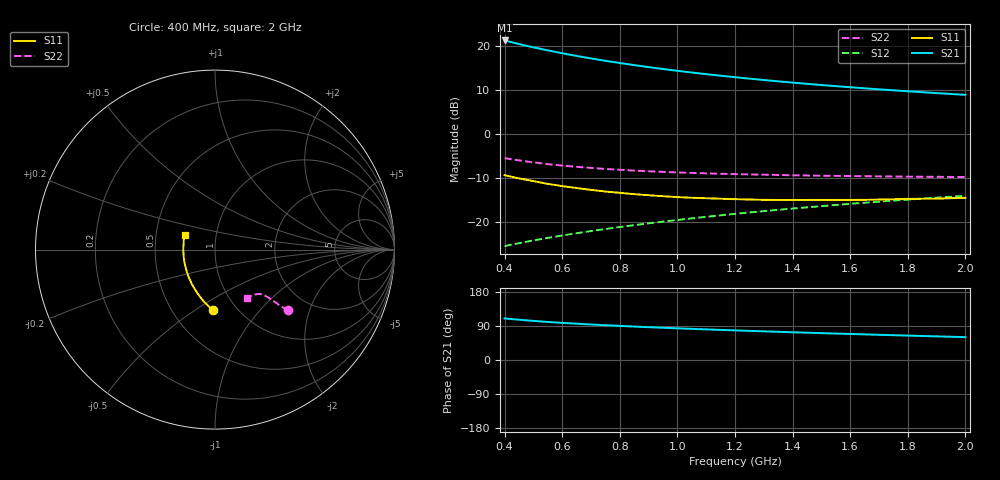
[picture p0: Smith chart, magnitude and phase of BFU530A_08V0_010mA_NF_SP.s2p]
! Filename:  P:\Prog\Test\Noise\ATS_data\Testdata_Net\06 Compressed Noise after Statistics\BFU530A_APG2013_33_A05_08p0V_010mA_NF_CM01_D.sf
! Date/Time: Tue 16/Apr/2013 15:11:01
! BFU530A_APG2013_33_A05_08p0V_1to25mA_NF_CM01_Bias5_R.sf
! Noise Parameter Data File
! BFU530A_APG2013_33_A05_08p0V_1to25mA_NF_CM01
! Date/time: Fri Apr 12 16:45:05 2013
! VAR V_out= 8.001000
! VAR I_out= 9.995000
! VAR V_in= 0.820500
! VAR I_in= 0.102910
! Device data file deembeded for feedlines and parallel
! Original file: \06 Compressed Noise after Statistics\BFU530A_APG2013_33_A05_08p0V_010mA_NF_CM01_R.sf
! Feed-files: PR017V01_150413_Feed1.s2p, PR017V01_150413_Feed2.s2p
! Parallel-file: PR017V01_150413_Par.s2p
# MHz S MA R 50
!  Freq-MHz  S11-mag  S11-arg  S21-mag  S21-arg  S12-mag  S12-arg  S22-mag  S22-arg
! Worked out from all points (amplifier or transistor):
!   37 points, 400 MHz to 2 GHz, reference 50 ohm
!   highest |S21| = 21.3 dB at 400 MHz (marker M1)
!   |S21| within 3 dB of that: start of sweep to 606.9 MHz
!   unconditionally stable (mu >= 1): 1.335 GHz to end of sweep
!   at 500 MHz: K = 0.80, MSG = 22.0 dB, |S12| = -24.3 dB
!   at 1.1 GHz: K = 0.98, MSG = 16.2 dB, |S12| = -18.9 dB
!   at 2 GHz: K = 1.01, MAG = 11.0 dB, |S12| = -14.1 dB
!   lowest NFmin = 0.76 dB at 433 MHz
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400  0.3384 -91.7  11.59 109.8  0.05265 65.0  0.5294 -39.6
420  0.3274 -94.2  11.16 108.3  0.05443 65.0  0.5163 -39.9
440  0.3163 -96.8  10.75 106.9  0.0561 65.1  0.5048 -40.1
480  0.2984 -101.5  10.01 104.4  0.05948 65.3  0.4836 -40.6
500  0.2896 -103.8  9.673 103.2  0.06122 65.4  0.4745 -40.8
550  0.2696 -109.5  8.942 100.4  0.06535 65.7  0.4523 -41.1
600  0.2544 -114.5  8.287 98.0  0.06966 66.0  0.4359 -41.3
650  0.2418 -119.4  7.727 95.8  0.07396 66.3  0.422 -41.6
700  0.2304 -124.1  7.235 93.7  0.07826 66.6  0.4098 -41.8
750  0.2207 -128.6  6.798 91.8  0.08259 66.9  0.399 -42.0
800  0.2134 -133.1  6.416 90.0  0.087 67.1  0.3905 -42.2
850  0.206 -137.5  6.072 88.3  0.09137 67.3  0.3821 -42.5
900  0.2003 -141.6  5.763 86.6  0.0958 67.4  0.3751 -42.8
950  0.1952 -145.5  5.484 85.1  0.1002 67.5  0.3695 -43.2
1050  0.1874 -153.0  5 82.2  0.1092 67.7  0.3595 -43.8
1150  0.1828 -160.3  4.598 79.4  0.1182 67.7  0.3513 -44.7
1200  0.1806 -163.6  4.422 78.1  0.1228 67.6  0.3485 -45.2
1350  0.1768 -173.0  3.968 74.4  0.1366 67.3  0.3408 -46.9
1500  0.177 178.1  3.604 70.9  0.1504 66.9  0.334 -48.7
1650  0.1775 170.4  3.307 67.6  0.1645 66.3  0.3299 -50.9
1750  0.1802 165.7  3.136 65.5  0.1737 65.9  0.3271 -52.3
2000  0.1872 155.1  2.785 60.4  0.1973 64.5  0.3231 -56.5
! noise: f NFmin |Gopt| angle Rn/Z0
400  0.8112  0.04272  177.9  0.0919
460  0.7758  0.04542  -179.5  0.0924
600  0.8757  0.0141  -145.4  0.1107
800  0.8488  0.07806  -176.9  0.0875
1000  0.8777  0.1036  175.7  0.0819
1200  0.9013  0.111  -172.1  0.0867
1400  0.9449  0.1308  -163  0.0847
1600  0.9537  0.1609  -159.8  0.0832
1800  0.9496  0.2034  -161.7  0.0727
2000  0.942  0.2231  -152.9  0.0799
